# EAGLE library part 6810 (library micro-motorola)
MICROCONTROLLER/MEMORY DEVICE
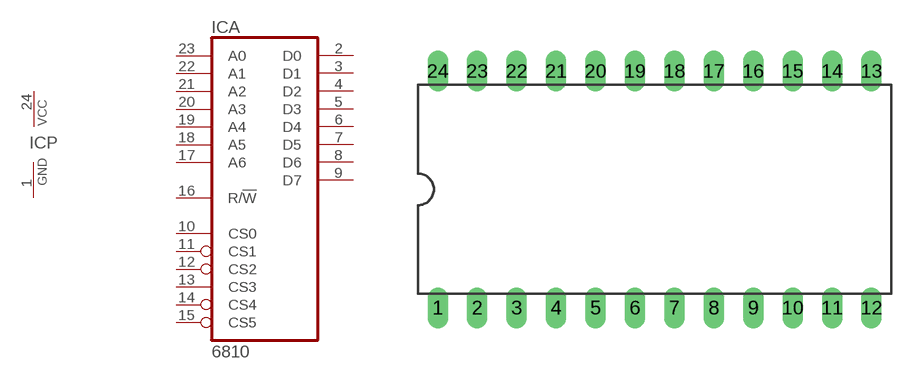
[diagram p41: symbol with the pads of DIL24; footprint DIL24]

Designator prefix IC; gates A=6810 P=PWRN

## 6810 (MF: NTE ELECTRONICS; MPN: NTE6810; OC_FARNELL: unknown; OC_NEWARK: 31C5319)  [DIL24]
1  P:GND  pwr
2  A:D0
3  A:D1
4  A:D2
5  A:D3
6  A:D4
7  A:D5
8  A:D6
9  A:D7
10  A:CS0  in
11  A:CS1  in
12  A:CS2  in
13  A:CS3  in
14  A:CS4  in
15  A:CS5  in
16  A:R/!W  in
17  A:A6  in
18  A:A5  in
19  A:A4  in
20  A:A3  in
21  A:A2  in
22  A:A1  in
23  A:A0  in
24  P:VCC  pwr

## Footprint DIL24 (pad centres in mm)
Dual In Line Package
drill 0.813 long: 1 -13.97,-7.62; 2 -11.43,-7.62; 3 -8.89,-7.62; 4 -6.35,-7.62; 5 -3.81,-7.62; 6 -1.27,-7.62; 7 1.27,-7.62; 8 3.81,-7.62; 9 6.35,-7.62; 10 8.89,-7.62; 11 11.43,-7.62; 12 13.97,-7.62; 13 13.97,7.62; 14 11.43,7.62; 15 8.89,7.62; 16 6.35,7.62; 17 3.81,7.62; 18 1.27,7.62; 19 -1.27,7.62; 20 -3.81,7.62; 21 -6.35,7.62; 22 -8.89,7.62; 23 -11.43,7.62; 24 -13.97,7.62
